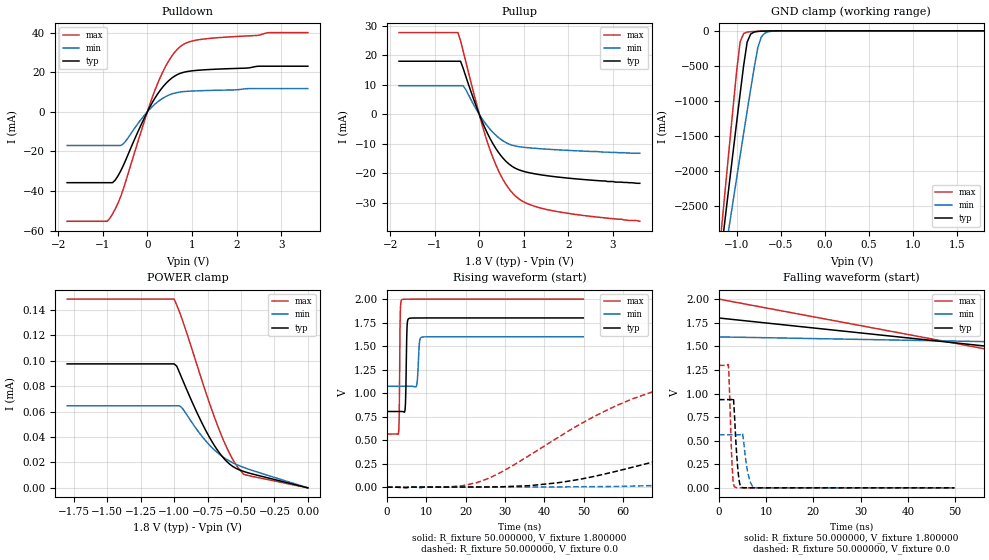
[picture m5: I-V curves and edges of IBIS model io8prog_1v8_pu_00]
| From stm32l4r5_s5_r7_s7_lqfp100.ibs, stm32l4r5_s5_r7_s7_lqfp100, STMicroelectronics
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|   Model io8prog_1v8_pu_00
[Model]  io8prog_1v8_pu_00
Model_type I/O
Polarity   Non-Inverting
Enable   Active-Low
Vinl =   0.540000V
Vinh =   1.260000V
Vmeas =  0.900000V
Cref =   100.000000nF
Rref =   1.000000k
Vref =   1.800000V
C_comp   2.197300pF   2.162700pF   2.264100pF
[Temperature Range]   25.000000   0.125000k   -40.000000
[Pullup Reference]   1.800000V   1.600000V   2.000000V
[Pulldown Reference]   0.0V   0.0V   0.0V
[POWER Clamp Reference]   1.800000V   1.600000V   2.000000V
[GND Clamp Reference]   0.0V   0.0V   0.0V
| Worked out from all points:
|   slope of the pulldown table from 0 to 0.27 V, typ, clamps not added: 26.2 ohm
|   slope of the pullup table from 0 to 0.27 V, typ, clamps not added: 30.1 ohm
|   GND clamp passes 1 mA (typ) near -0.58 V on its own axis
|   rising waveform, R_fixture 50.000000, V_fixture 1.800000: 20-80 % time 248ps typ, 382ps min, 183ps max; typ from 0.805 V to 1.8 V
|   rising waveform, R_fixture 50.000000, V_fixture 0.0: 20-80 % time 65.3ns typ, 116ns min, 36.2ns max; typ from 0.001 V to 0.935 V
|   falling waveform, R_fixture 50.000000, V_fixture 1.800000: 20-80 % time 116ns typ, 164ns min, 91.9ns max; typ from 1.8 V to 0.805 V
|   falling waveform, R_fixture 50.000000, V_fixture 0.0: 20-80 % time 712ps typ, 1.01ns min, 547ps max; typ from 0.935 V to 0.001 V
[Pulldown]
|Voltage   I(typ)   I(min)   I(max)
-1.8V     -35.82mA   -17.03mA   -55.35mA
-900mV    -35.82mA   -17.03mA   -55.35mA
-840mV    -35.82mA   -17.03mA   -53.76mA
-720mV    -34.49mA   -17.03mA   -49.08mA
-540mV    -27.18mA   -16.22mA   -39.07mA
-60mV     -2.756mA   -1.584mA   -4.226mA
240mV     9.353mA    5.171mA    14.85mA
480mV     15.75mA    8.427mA    25.77mA
720mV     19.29mA    9.947mA    32.62mA
960mV     20.57mA    10.43mA    35.5mA
1.32V     21.27mA    10.74mA    36.91mA
3.6V      23.03mA    11.73mA    40.04mA
[Pullup]
|Voltage   I(typ)   I(min)   I(max)
-1.8V     18.05mA    9.741mA    27.78mA
-480mV    18.05mA    9.741mA    27.78mA
-420mV    18.05mA    9.741mA    25.03mA
-360mV    15.57mA    9.741mA    21.38mA
60mV      -2.268mA   -1.401mA   -3.341mA
240mV     -8.143mA   -5.004mA   -12mA
360mV     -11.31mA   -6.914mA   -16.72mA
540mV     -15mA      -9.056mA   -22.31mA
840mV     -18.52mA   -10.83mA   -28.11mA
1.14V     -19.87mA   -11.38mA   -30.67mA
1.62V     -21.02mA   -11.91mA   -32.63mA
3.6V      -23.4mA    -13.2mA    -36.3mA
[GND_clamp]
|Voltage   I(typ)   I(min)   I(max)
-1.8V     -9.861A    -8.8A      -9.626A
-1.16V    -3.004A    -3.417A    -2.68A
-1.12V    -2.579A    -3.088A    -2.15A
-1.08V    -2.155A    -2.76A     -1.623A
-1V       -1.315A    -2.108A    -586.3mA
-960mV    -900.6mA   -1.784A    -158.3mA
-920mV    -496.8mA   -1.462A    -39.39mA
-880mV    -160.5mA   -1.144A    -17.82mA
-840mV    -45.92mA   -830.3mA   -12.52mA
-760mV    -8.262mA   -243mA     -7.547mA
-680mV    -3.389mA   -33.05mA   -3.833mA
1.8V      0A         0A         0A
[POWER_clamp]
|Voltage   I(typ)   I(min)   I(max)
-1.8V     97.61uA    64.61uA    148.6uA
-1V       97.61uA    64.61uA    148.6uA
-980mV    95.77uA    64.61uA    143.9uA
-960mV    90.85uA    64.61uA    138.6uA
-940mV    85.82uA    62.87uA    132.7uA
-820mV    57.18uA    44.44uA    93.74uA
-720mV    36.98uA    32uA       61.96uA
-620mV    22.23uA    23.29uA    34.8uA
-560mV    16.76uA    19.67uA    22.06uA
-520mV    14.49uA    17.74uA    15.63uA
-480mV    12.91uA    16.08uA    10.62uA
0V        0A         0A         0A
[Ramp]
| variable   typ   min   max
dV/dt_r  0.56074/65.15328n   0.33715/0.11613u   0.77863/36.11629n
dV/dt_f  0.59675/66.14092n   0.31608/0.11580u   0.86035/34.94520n
R_load = 50.000000
[Rising Waveform]
R_fixture= 50.000000
V_fixture= 1.800000
V_fixture_min= 1.600000
V_fixture_max= 2.000000
|time   V(typ)   V(min)   V(max)
0s        805.4mV    1.073V     566.1mV
2.903ns   805.4mV    1.073V     567.4mV
3.103ns   805.5mV    1.073V     741.6mV
3.403ns   805.4mV    1.073V     1.899V
3.804ns   805.2mV    1.073V     1.994V
4.605ns   829.2mV    1.073V     1.999V
5.105ns   1.72V      1.073V     1.999V
5.606ns   1.795V     1.073V     2V
8.809ns   1.8V       1.595V     2V
49.85ns   1.8V       1.6V       2V
[Rising Waveform]
R_fixture= 50.000000
V_fixture= 0.0
V_fixture_min= 0.0
V_fixture_max= 0.0
|time   V(typ)   V(min)   V(max)
0s        725.1uV    1.151mV    481.9uV
24.02ns   2.96mV     2.594mV    66.56mV
43.24ns   46.77mV    3.569mV    524.2mV
55.26ns   140.5mV    7.488mV    807.7mV
73.27ns   329.9mV    23.85mV    1.087V
109.3ns   656.2mV    119.8mV    1.262V
140.5ns   809.8mV    231.7mV    1.288V
171.8ns   879.9mV    333.9mV    1.295V
261.9ns   930.7mV    500.9mV    1.298V
598.2ns   935.3mV    563.1mV    1.298V
[Falling Waveform]
R_fixture= 50.000000
V_fixture= 1.800000
V_fixture_min= 1.600000
V_fixture_max= 2.000000
|time   V(typ)   V(min)   V(max)
0s        1.8V       1.6V       2V
150.2ns   1.008V     1.466V     594.8mV
300.3ns   818.5mV    1.138V     566.8mV
450.5ns   806.4mV    1.085V     566.1mV
750.8ns   805.4mV    1.074V     566.1mV
14.86us   805.4mV    1.073V     566.1mV
[Falling Waveform]
R_fixture= 50.000000
V_fixture= 0.0
V_fixture_min= 0.0
V_fixture_max= 0.0
|time   V(typ)   V(min)   V(max)
0s        935.3mV    563.1mV    1.298V
2.002ns   935.5mV    563.1mV    1.304V
2.803ns   939.3mV    563.2mV    229.2mV
3.103ns   929.5mV    563.3mV    39.8mV
3.403ns   667.7mV    563.3mV    8.256mV
4.104ns   151.9mV    563mV      1.962mV
4.805ns   5.628mV    576.1mV    1.506mV
6.306ns   870.4uV    119.8mV    1.426mV
7.508ns   746.4uV    3.798mV    1.412mV
49.85ns   725.1uV    1.151mV    481.9uV
